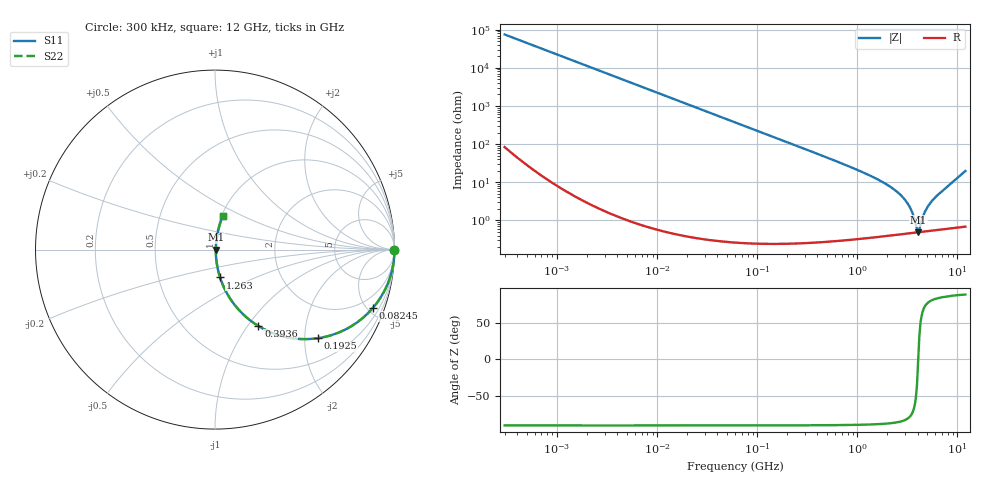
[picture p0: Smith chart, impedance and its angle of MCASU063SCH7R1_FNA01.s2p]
! MCASU063SCH7R1_FNA01  S-PARAMETER MODEL  ( General Type )
! Model Generated by TAIYO YUDEN Corporation (http://www.ty-top.com)
! Version 1.0
! TAIYO YUDEN Control No. 130801
! Copyright(c) 2013 TAIYO YUDEN CO.,LTD. All Rights Reserved.
! Product Description (link to TY-COMPAS)
! https://ds.yuden.co.jp/TYCOMPAS/or/detail?pn=MCASU063SCH7R1DFNA01&u=M
! Products Name : Multilayer Ceramic Capacitors
! Characteristics :
!  Capacitance : 7.1 pF , Rated Voltage : 50V , TCC : CH / C0H
!  Case Size : 0.6 x 0.3 / 0.024 x 0.012 [mm/inch] , Thickness : 0.3 / 0.012 [mm/inch]
!  (Conditions: Temperature = 25 degC , DC Bias Current/Voltage = 0A / 0V)
! External Node Assignments :
!  1  o---| |---o  2
! GND o---------o GND
! Frequency Range : 0.3MHz  -  12000MHz  [ 401 STEP ]
# MHz S RI R 50
! Freq[MHz].  S11 Real  S11 Imag  S21 Real  S21 Imag  S12 Real  S12 Imag  S22 Real  S22 Imag
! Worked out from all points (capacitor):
!   401 points, 300 kHz to 12 GHz, reference 50 ohm
!   read as one part in series: C = 7.12 pF near 316.3 kHz
!   lowest |Z| = 488 mohm at 4.05 GHz (marker M1)
!   series resonance near 4.053 GHz, so ESL is about 220 pH
!   S11 on the Smith chart (normalised r, x): 300 kHz: open; 82.45 MHz: 1.00, -5.42; 192.5 MHz: 1.00, -2.32; 393.6 MHz: 1.01, -1.13; 1.263 GHz: 1.01, -0.32; 12 GHz: 1.01, +0.39
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0.3  1 -0.00134  3.3e-06 0.00134  3.3e-06 0.00134  1 -0.00134
1.769972  0.9999 -0.00791  6.48e-05 0.00791  6.48e-05 0.00791  0.9999 -0.00791
10.44266  0.9978 -0.0466  0.00219 0.0466  0.00219 0.0466  0.9978 -0.0466
27.10171  0.9855 -0.1194  0.0145 0.1194  0.0145 0.1194  0.9855 -0.1194
60  0.9327 -0.2503  0.0673 0.2503  0.0673 0.2503  0.9327 -0.2503
82.45425  0.88 -0.3245  0.12 0.3245  0.12 0.3245  0.88 -0.3245
125.9782  0.7584 -0.4274  0.2416 0.4274  0.2416 0.4274  0.7584 -0.4274
192.4766  0.5732 -0.4936  0.4268 0.4936  0.4268 0.4936  0.5732 -0.4936
353.9943  0.2829 -0.4484  0.7171 0.4484  0.7171 0.4484  0.2829 -0.4484
393.5654  0.2416 -0.4257  0.7584 0.4257  0.7584 0.4257  0.2416 -0.4257
668.5285  0.0979 -0.2927  0.9021 0.2927  0.9021 0.2927  0.0979 -0.2927
1262.535  0.0281 -0.155  0.9719 0.155  0.9719 0.155  0.0281 -0.155
2088.533  0.0101 -0.0777  0.9899 0.0777  0.9899 0.0777  0.0101 -0.0777
2650.866  0.00657 -0.048  0.9934 0.048  0.9934 0.048  0.00657 -0.048
3107.553  0.00535 -0.0296  0.9946 0.0296  0.9946 0.0296  0.00535 -0.0296
3454.93  0.00494 -0.0178  0.9951 0.0178  0.9951 0.0178  0.00494 -0.0178
3841.137  0.00482 -0.0062  0.9952 0.0062  0.9952 0.0062  0.00482 -0.0062
4050.141  0.00486 -7.46e-05  0.9951 7.46e-05  0.9951 7.46e-05  0.00486 -7.46e-05
4270.516  0.00498 0.00575  0.995 -0.00575  0.995 -0.00575  0.00498 0.00575
4875.354  0.0055 0.0186  0.9945 -0.0186  0.9945 -0.0186  0.0055 0.0186
5565.855  0.00638 0.0316  0.9936 -0.0316  0.9936 -0.0316  0.00638 0.0316
12000  0.0434 0.1872  0.9566 -0.1872  0.9566 -0.1872  0.0434 0.1872
